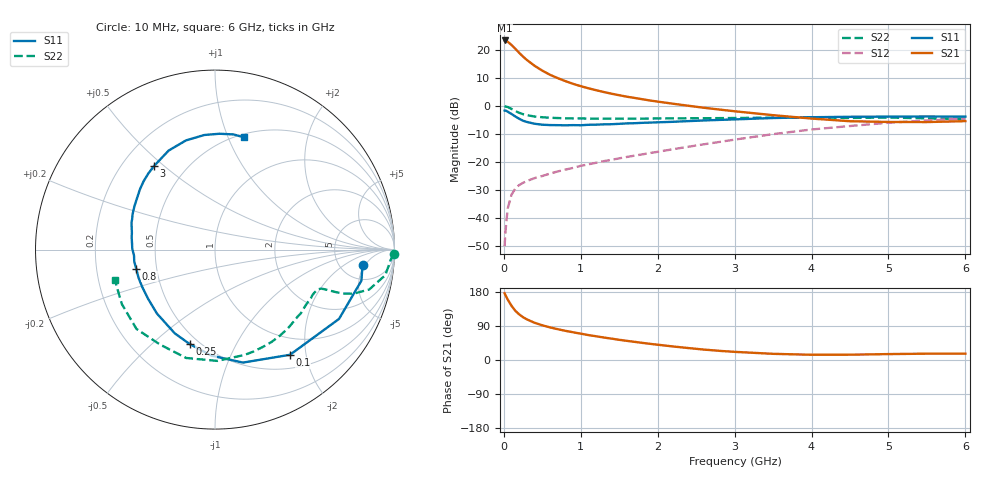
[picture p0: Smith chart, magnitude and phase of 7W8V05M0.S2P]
! Infineon Technologies  Discrete & RF Semiconductors
! BFS17W
! Si NPN RF Bipolar Junction Transistor in SOT323
! VCE = 8 V  IC = 5 mA
! Common Emitter S-Parameters:  August  1999
# GHz  S  MA  R  50
!  f  S11  S21  S12  S22
! GHz  MAG  ANG  MAG  ANG  MAG  ANG  MAG  ANG
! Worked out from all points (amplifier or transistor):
!   36 points, 10 MHz to 6 GHz, reference 50 ohm
!   highest |S21| = 23.5 dB at 10 MHz (marker M1)
!   |S21| within 3 dB of that: start of sweep to 149.9 MHz
!   unconditionally stable (mu >= 1): 584.9 MHz to 2.367 GHz; 5.214 GHz to end of sweep
!   at 250 MHz: K = 0.57, MSG = 22.6 dB, |S12| = -27.5 dB
!   at 1.4 GHz: K = 1.21, MAG = 9.1 dB, |S12| = -19.3 dB
!   at 6 GHz: K = 1.05, MAG = -1.8 dB, |S12| = -4.5 dB
!   S11 on the Smith chart (normalised r, x): 10 MHz: 8.16, -4.38; 100 MHz: 0.71, -1.72; 250 MHz: 0.45, -0.67; 800 MHz: 0.38, -0.10; 3 GHz: 0.33, +0.46; 6 GHz: 0.53, +1.15
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0.01  0.8266 -5.9  14.9 176.1  0.0031 79.3  0.9967 -1.3
0.02  0.8338 -12.0  14.78 171.6  0.0054 90.6  0.9794 -3.5
0.05  0.7916 -29.2  14.15 159.6  0.0146 76.1  0.96 -8.5
0.1  0.7197 -54.5  12.36 143.0  0.0259 65.1  0.8875 -14.5
0.15  0.6485 -76.1  10.54 129.7  0.0334 57.0  0.8113 -17.6
0.2  0.5912 -91.9  8.944 120.3  0.0386 53.7  0.7551 -18.9
0.25  0.5448 -105.0  7.654 112.9  0.0422 51.2  0.7134 -19.4
0.3  0.5178 -115.6  6.654 107.2  0.0455 50.8  0.6852 -19.6
0.4  0.4813 -132.2  5.24 98.2  0.0512 50.9  0.6481 -19.9
0.5  0.4625 -143.8  4.294 91.6  0.0559 52.8  0.6287 -20.2
0.6  0.4558 -152.9  3.624 86.0  0.0617 54.5  0.6166 -21.0
0.8  0.4516 -166.4  2.789 77.0  0.0727 57.9  0.6029 -23.6
0.9  0.4548 -171.6  2.494 73.2  0.0781 59.6  0.5989 -25.1
1.1  0.461 179.4  2.075 65.7  0.0904 61.9  0.5958 -28.5
1.3  0.4695 171.5  1.78 59.3  0.1032 64.1  0.5928 -32.7
1.6  0.4887 162.2  1.467 50.5  0.1225 66.5  0.5926 -39.0
2.2  0.5217 146.1  1.098 35.7  0.1686 70.4  0.6009 -53.4
3  0.5762 126.2  0.805 21.5  0.2501 70.4  0.6095 -74.3
3.5  0.6092 115.1  0.685 16.3  0.3138 67.4  0.6202 -88.8
4.5  0.6413 95.3  0.534 14.0  0.4382 55.8  0.6112 -120.1
5.5  0.6499 80.9  0.516 16.7  0.5503 42.5  0.6012 -149.7
6  0.646 75.4  0.536 16.7  0.595 35.9  0.5833 -162.9
